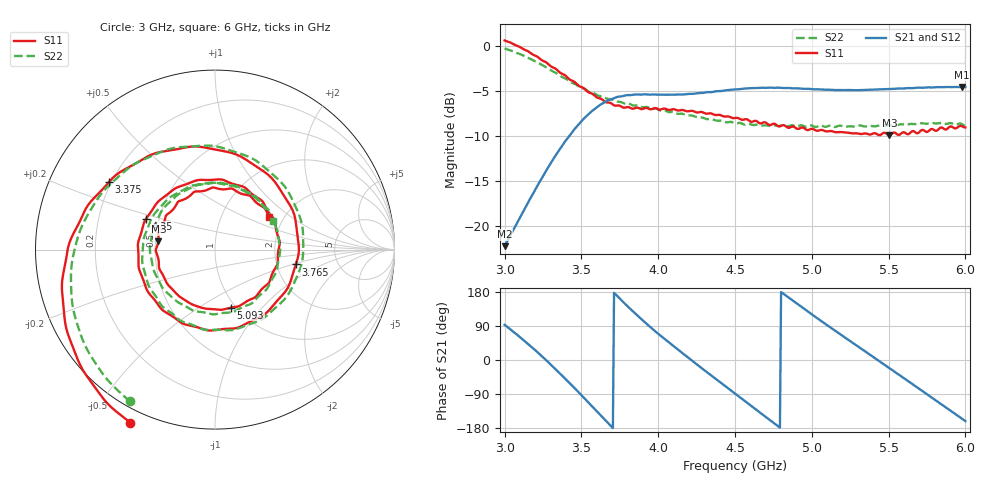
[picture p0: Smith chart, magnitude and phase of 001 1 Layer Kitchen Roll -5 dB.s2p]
!  04/11/2025  13:29:57
! Ref Plane: 0.000 mm
# MHZ S MA R  50
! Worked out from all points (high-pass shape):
!   401 points, 3 GHz to 6 GHz, reference 50 ohm
!   highest |S21| = -4.55 dB at 5.978 GHz (marker M1); lowest = -22.2 dB at 3 GHz (marker M2)
!   |S21| within 3 dB of the highest: 3.548 GHz to end of sweep
!   lowest |S11| = -9.9 dB at 5.505 GHz (marker M3), VSWR 1.94, Z = 25.9 + j2.69 ohm
!   |S11| at or under -10 dB: nowhere
!   |S22| runs from -9.0 to -0.3 dB; largest |S21 - S12| = 0.01
!   S11 on the Smith chart (normalised r, x): 3 GHz: -0.05, -0.62; 3.375 GHz: 0.19, +0.28; 3.765 GHz: 2.56, -0.54; 4.35 GHz: 0.42, +0.18; 5.093 GHz: 0.95, -0.69; 6 GHz: 1.69, +0.70
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3000  1.073 -116.1  0.07738 92.8  0.07798 93.5  0.9696 -119.3
3195  0.8869 -163.5  0.1568 27.5  0.1575 27.9  0.8244 -166.7
3375  0.7001 147.3  0.2794 -41.2  0.28 -40.9  0.6721 142.1
3502.5  0.5907 104.4  0.3842 -93.8  0.3844 -93.5  0.584 98.1
3645  0.4968 44.8  0.483 -154.5  0.4856 -154.1  0.5211 39.1
3765  0.4577 -10.4  0.5258 155.8  0.528 156.4  0.4852 -13.8
3885  0.4475 -60.2  0.5365 109.8  0.5382 110.5  0.4614 -62.0
4005  0.444 -101.9  0.5365 67.8  0.5364 68.5  0.4411 -103.7
4185  0.4341 -156.0  0.5403 9.7  0.5416 10.1  0.4125 -159.1
4350  0.4205 155.7  0.5547 -42.4  0.556 -41.7  0.3927 150.3
4500  0.3983 108.5  0.5743 -88.8  0.5767 -88.3  0.3724 101.6
4620  0.3818 69.3  0.584 -125.9  0.5856 -125.4  0.3639 61.9
4762.5  0.3683 23.9  0.5861 -169.4  0.5876 -168.8  0.3619 14.8
4875  0.3575 -12.4  0.5814 156.9  0.583 157.5  0.3627 -20.7
5002.5  0.347 -49.6  0.5754 119.8  0.5768 120.3  0.3611 -58.0
5092.5  0.3356 -74.6  0.5717 94.0  0.5735 94.6  0.3557 -83.8
5325  0.3246 -137.8  0.569 28.9  0.5713 29.4  0.3606 -145.7
5505  0.3186 171.6  0.5768 -21.3  0.5795 -20.9  0.3637 164.1
5745  0.3333 102.7  0.5889 -88.9  0.5917 -88.4  0.3699 96.7
5857.5  0.3483 71.2  0.5909 -120.7  0.5939 -120.1  0.371 66.2
5977.5  0.3587 37.6  0.5921 -154.7  0.595 -154.1  0.3684 33.4
6000  0.353 30.7  0.5917 -161.3  0.5939 -160.7  0.3614 26.3
